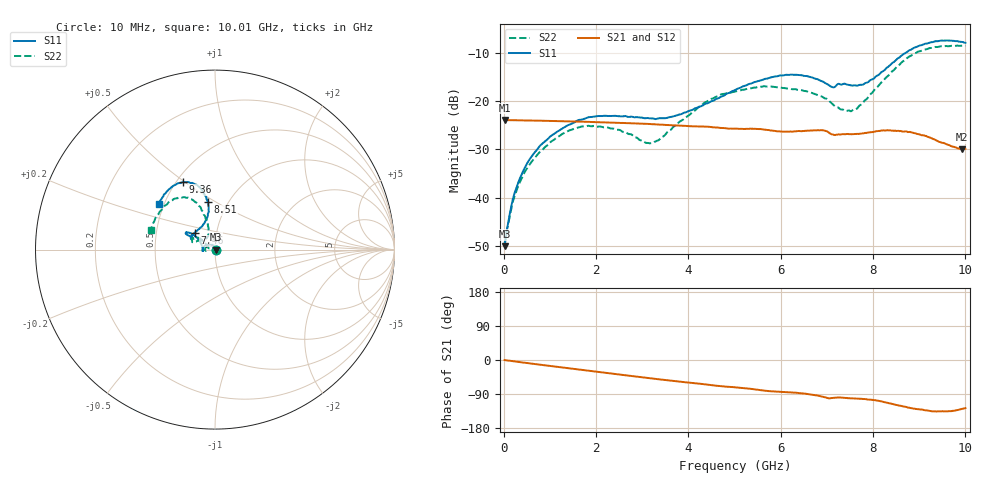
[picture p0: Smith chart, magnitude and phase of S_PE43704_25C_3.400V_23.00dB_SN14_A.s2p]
! Device ID: PE43704
! Dir: z:\PE43704\PE43704_Char_1_20130516\PE43704\AMB\3p400V\23p00dB
! Serial: 14
! Insertion: A
! Impedance: 50 ohm
! Temp: Amb
! VDD: 3.400V
! Attenuation Step: 23.00dB
! IDD: 1.140390e-01mA
#  Hz  S  RI  R  50
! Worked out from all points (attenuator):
!   401 points, 10 MHz to 10.01 GHz, reference 50 ohm
!   highest |S21| = -23.92 dB at 10 MHz (marker M1); lowest = -29.9 dB at 9.935 GHz (marker M2)
!   lowest |S11| = -50.0 dB at 10 MHz (marker M3), VSWR 1.01, Z = 50.3 + j0.0429 ohm
!   |S11| at or under -10 dB: start of sweep to 8.719 GHz
!   |S22| runs from -49.4 to -8.5 dB; largest |S21 - S12| = 0.00078
!   S11 on the Smith chart (normalised r, x): 10 MHz: 1.01, +0.00; 7.46 GHz: 0.78, +0.15; 8.51 GHz: 0.81, +0.46; 9.36 GHz: 0.54, +0.49; 10.01 GHz: 0.47, +0.28
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1e7  0.00313 0.000426  0.0637 -0.000225  0.0637 -0.000199  0.00337 0.000396
1.6e8  0.00279 0.00788  0.0634 -0.00297  0.0634 -0.00295  0.00312 0.00722
2.35e8  0.00134 0.0114  0.0632 -0.00429  0.0633 -0.00428  0.00183 0.0105
5.35e8  -0.00719 0.0232  0.0624 -0.00943  0.0624 -0.00934  -0.00644 0.0205
1.085e9  -0.0351 0.0294  0.0596 -0.0183  0.0597 -0.0183  -0.0321 0.0237
1.685e9  -0.0626 0.0157  0.055 -0.0271  0.055 -0.027  -0.0542 0.00759
2.485e9  -0.0695 -0.00589  0.0469 -0.0368  0.0469 -0.0368  -0.05 -0.00686
3.11e9  -0.0666 -0.00598  0.0394 -0.0427  0.0395 -0.0427  -0.0366 0.0048
3.36e9  -0.0665 -9.96e-05  0.036 -0.0444  0.036 -0.0444  -0.0373 0.0137
4.385e9  -0.0839 0.0437  0.0233 -0.0491  0.0233 -0.0492  -0.0793 0.058
5.01e9  -0.1079 0.0726  0.0158 -0.0494  0.016 -0.0493  -0.1091 0.0624
5.96e9  -0.1556 0.096  0.00529 -0.0485  0.00564 -0.0484  -0.1279 0.0525
6.685e9  -0.1555 0.0824  -0.00141 -0.0496  -0.00122 -0.0495  -0.1132 0.0436
7.11e9  -0.1248 0.0642  -0.00824 -0.0446  -0.00824 -0.0446  -0.0797 0.0521
7.46e9  -0.1142 0.0938  -0.00856 -0.0449  -0.00831 -0.0449  -0.0511 0.0614
7.835e9  -0.0674 0.1379  -0.0107 -0.0457  -0.0105 -0.0456  -0.0357 0.0961
8.36e9  -0.0355 0.2295  -0.0204 -0.0454  -0.0204 -0.0455  -0.0537 0.1808
8.51e9  -0.0385 0.2647  -0.0236 -0.0431  -0.0232 -0.0434  -0.0677 0.2127
8.935e9  -0.089 0.3504  -0.0293 -0.0359  -0.0293 -0.0357  -0.1384 0.283
9.36e9  -0.1791 0.3763  -0.0283 -0.0277  -0.0286 -0.0275  -0.2312 0.281
9.935e9  -0.3015 0.2782  -0.02 -0.0247  -0.0203 -0.0248  -0.3478 0.1401
1.001e10  -0.3129 0.2515  -0.0193 -0.0256  -0.0197 -0.0253  -0.3572 0.1113
